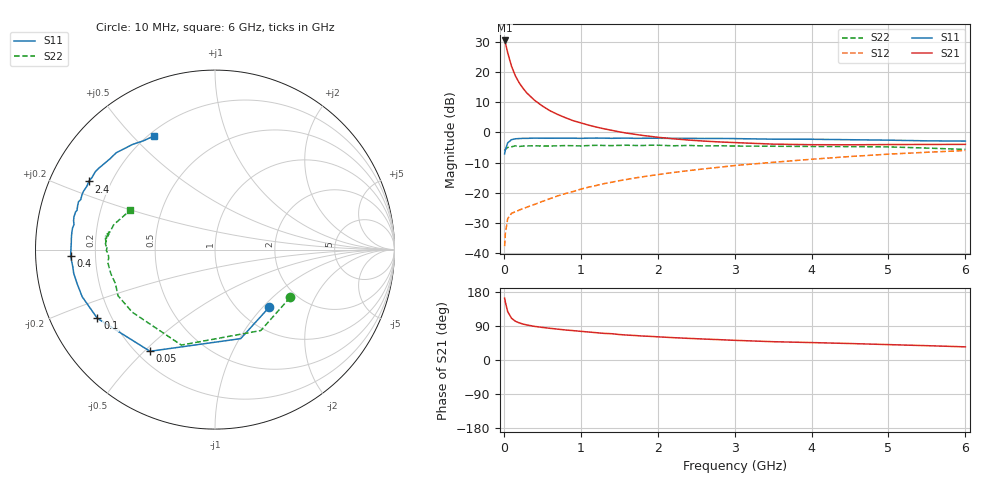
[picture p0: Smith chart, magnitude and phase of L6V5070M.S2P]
!  INFINEON TECHNOLOGIES Small Signal Semiconductors
! BFR380L3 , Si-NPN RF-Transistor in TSLP-3-1
!  Vce=0.5 V,  Ic=70 mA
! Common Emitter S-Parameters:  07. March 2005
#  GHz  S  MA  R  50
! f  S11  S21  S12  S22
! GHz  Mag  Ang  Mag  Ang  Mag  Ang  Mag  Ang
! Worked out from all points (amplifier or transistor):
!   36 points, 10 MHz to 6 GHz, reference 50 ohm
!   highest |S21| = 30.6 dB at 10 MHz (marker M1)
!   |S21| within 3 dB of that: start of sweep to 40.18 MHz
!   unconditionally stable (mu >= 1): 521.8 MHz to end of sweep
!   at 250 MHz: K = 0.68, MSG = 20.0 dB, |S12| = -25.3 dB
!   at 1.4 GHz: K = 1.20, MAG = 5.9 dB, |S12| = -16.6 dB
!   at 6 GHz: K = 1.07, MAG = -0.6 dB, |S12| = -6.0 dB
!   S11 on the Smith chart (normalised r, x): 10 MHz: 1.37, -1.09; 50 MHz: 0.25, -0.52; 100 MHz: 0.15, -0.27; 400 MHz: 0.11, -0.02; 2.4 GHz: 0.12, +0.25; 6 GHz: 0.22, +0.58
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0.01  0.4406 -46.6  33.78 163.1  0.0129 52.4  0.4964 -32.5
0.02  0.5163 -73.9  30.72 152.6  0.021 53.4  0.518 -60.5
0.05  0.6724 -122.6  21.17 127.6  0.0369 39.5  0.564 -109.4
0.1  0.7593 -149.7  12.57 110.1  0.0454 30.9  0.5781 -142.9
0.15  0.7852 -160.5  8.723 102.3  0.0481 30.7  0.5985 -154.6
0.2  0.7915 -166.2  6.669 97.9  0.0513 32.9  0.586 -161.1
0.25  0.7982 -170.5  5.409 94.7  0.0543 35.3  0.5945 -166.4
0.3  0.7979 -172.9  4.514 92.5  0.0573 38.0  0.5969 -168.3
0.4  0.8053 -177.4  3.417 88.7  0.0639 43.1  0.6015 -173.2
0.5  0.8024 179.4  2.756 86.0  0.0714 47.2  0.5941 -175.5
0.6  0.8016 177.3  2.294 83.6  0.0794 50.1  0.5946 -176.8
0.7  0.8027 175.6  1.991 81.4  0.0882 52.9  0.6 -178.5
0.9  0.8028 171.3  1.571 77.5  0.1043 56.7  0.602 179.1
1.1  0.8041 168.5  1.325 73.9  0.1233 58.7  0.6063 178.3
1.3  0.8048 164.9  1.152 70.3  0.1408 59.4  0.6075 175.6
1.6  0.8058 160.7  0.974 65.8  0.1659 60.0  0.6135 174.1
2.2  0.7965 153.8  0.786 59.0  0.2161 59.9  0.6006 172.8
2.4  0.7989 151.6  0.748 57.1  0.2321 59.9  0.6088 171.2
3.5  0.7733 139.1  0.64 48.3  0.3192 56.1  0.5898 169.2
4.5  0.7574 132.3  0.624 43.5  0.3982 52.1  0.5827 166.6
5.5  0.7257 123.4  0.632 37.8  0.469 46.0  0.55 161.3
6  0.7187 118.3  0.634 34.7  0.5006 43.2  0.5224 155.3
